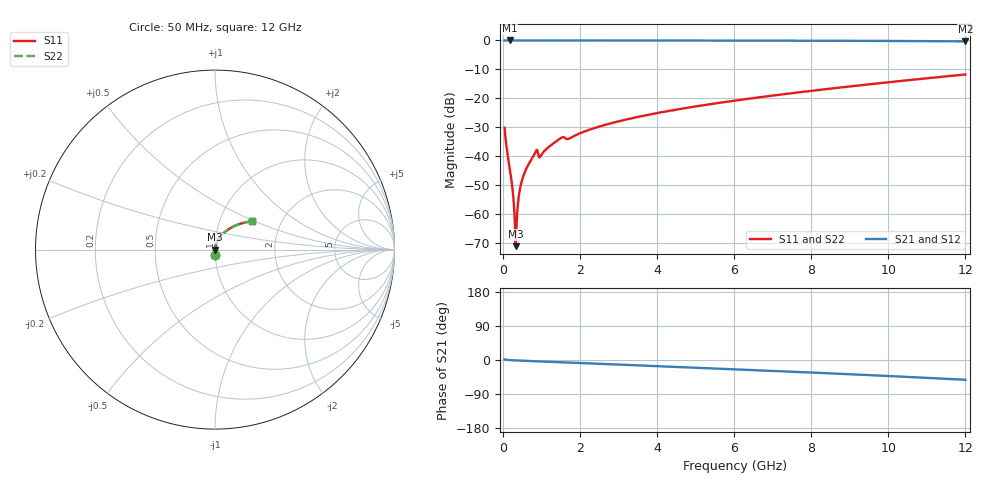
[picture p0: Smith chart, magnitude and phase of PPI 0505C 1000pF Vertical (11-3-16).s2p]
# GHz S MA R 50
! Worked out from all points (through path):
!   1601 points, 50 MHz to 12 GHz, reference 50 ohm
!   highest |S21| = 0.00 dB at 177 MHz (marker M1); lowest = -0.3 dB at 12 GHz (marker M2)
!   group delay of S21, straight-line fit = 12 ps
!   lowest |S11| = -71.1 dB at 341.3 MHz (marker M3), VSWR 1.00, Z = 50 + j0.00666 ohm
!   |S11| at or under -10 dB: start of sweep to end of sweep
!   |S22| runs from -71.1 to -11.8 dB; largest |S21 - S12| = 0
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0.05  0.0311 -88.1  0.9993 1.6  0.9993 1.6  0.0311 -88.1
0.1769688  0.006548 -88.2  0.9997 -0.2  0.9997 -0.2  0.006548 -88.2
0.2441875  0.003147 -86.1  0.9997 -0.6  0.9997 -0.6  0.003147 -86.1
0.2964688  0.001287 -79.3  0.9997 -0.9  0.9997 -0.9  0.001287 -79.3
0.318875  0.0006286 -66.1  0.9997 -1.0  0.9997 -1.0  0.0006286 -66.1
0.3412812  0.0002798 13.8  0.9997 -1.1  0.9997 -1.1  0.0002798 13.8
0.378625  0.001094 73.9  0.9997 -1.3  0.9997 -1.3  0.001094 73.9
0.438375  0.002498 81.7  0.9997 -1.6  0.9997 -1.6  0.002498 81.7
0.5130625  0.004101 83.7  0.9996 -1.9  0.9996 -1.9  0.004101 83.7
0.6250938  0.006346 84.4  0.9996 -2.4  0.9996 -2.4  0.006346 84.4
0.8416875  0.01144 80.6  0.9987 -3.4  0.9987 -3.4  0.01144 80.6
0.9835938  0.01006 77.4  0.9983 -3.7  0.9983 -3.7  0.01006 77.4
1.177781  0.01417 82.8  0.9992 -4.6  0.9992 -4.6  0.01417 82.8
1.506406  0.02059 78.8  0.9978 -6.0  0.9978 -6.0  0.02059 78.8
1.715531  0.02003 76.6  0.9973 -6.7  0.9973 -6.7  0.02003 76.6
2.044156  0.02553 80.1  0.9987 -8.0  0.9987 -8.0  0.02553 80.1
2.873187  0.03807 77.6  0.9984 -11.4  0.9984 -11.4  0.03807 77.6
4.038312  0.05618 73.1  0.9975 -16.1  0.9975 -16.1  0.05618 73.1
6.025  0.09145 65.1  0.9946 -24.4  0.9946 -24.4  0.09145 65.1
8.019156  0.1351 56.5  0.9894 -33.1  0.9894 -33.1  0.1351 56.5
10.01331  0.19 47.4  0.98 -42.3  0.98 -42.3  0.19 47.4
12  0.2582 37.6  0.964 -52.2  0.964 -52.2  0.2582 37.6
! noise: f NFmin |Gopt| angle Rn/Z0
0.05  0.0002881  0.8212  0.1957  0.0003378
1.372  0.003404  0.6288  4.3  0.001717
2.701  0.004461  0.4909  8.131  0.001498
4.031  0.005714  0.4326  11.7  0.001646
5.36  0.007002  0.4015  15.06  0.001861
6.682  0.008286  0.3829  18.19  0.002095
8.012  0.009605  0.3728  21.14  0.002356
9.341  0.01098  0.3697  23.94  0.002653
10.67  0.01244  0.3725  26.63  0.003
12  0.01401  0.3806  29.27  0.003413
